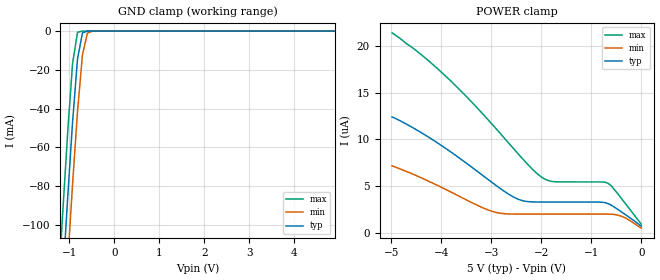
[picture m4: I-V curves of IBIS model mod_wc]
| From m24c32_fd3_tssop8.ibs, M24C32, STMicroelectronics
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|   Model mod_wc
[Model]   mod_wc
Model_type Input
Vinl   =   1.500V
Vinh   =   3.500V
C_comp   1.763pF   1.683pF   1.933pF
[Temperature Range]   25.0000   85.0000   -40.0000
[Voltage Range]   5.0000V   4.5000V   5.5000V
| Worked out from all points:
|   GND clamp passes 1 mA (typ) near -0.71 V on its own axis
[GND_clamp]
|Voltage   I(typ)   I(min)   I(max)
-5V       -1.733A    -1.764A    -1.703A
-1.26V    -171.7mA   -205.6mA   -137.3mA
-1.15V    -128.4mA   -162.2mA   -94.06mA
-1.04V    -86.41mA   -119.8mA   -52.72mA
-930mV    -46.94mA   -79.03mA   -16.7mA
-820mV    -14.34mA   -41.51mA   -622.7uA
-710mV    -879.9uA   -12.25mA   -4.426uA
-600mV    -18.76uA   -1.026mA   -29.45nA
-490mV    -372.8nA   -42.05uA   -196.9pA
4.9V      10.41pA    50.62pA    10.07pA
[POWER_clamp]
|Voltage   I(typ)   I(min)   I(max)
-4.98V    12.41uA    7.179uA    21.39uA
-4.5V     11.06uA    6.145uA    19.5uA
-4.02V    9.447uA    4.953uA    17.32uA
-3V       5.473uA    2.353uA    11.74uA
-2.46V    3.612uA    2.025uA    8.46uA
-2.04V    3.315uA    2.022uA    6.163uA
-1.92V    3.313uA    2.021uA    5.738uA
-1.74V    3.312uA    2.021uA    5.49uA
-840mV    3.31uA     2.02uA     5.46uA
-660mV    3.133uA    2.02uA     5.304uA
-360mV    2.122uA    1.721uA    3.437uA
0V        730nA      520.1nA    955.4nA
